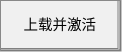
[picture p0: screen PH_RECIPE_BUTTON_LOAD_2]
VISUALIZATION PH_RECIPE_BUTTON_LOAD_2  // 122x52
VAR_IN_OUT
	RECIPE_CTRL_V2 : ST_RecipeCtrl_2;
END_VAR
    Button (0,0 120x50), "上载并激活", input disabled if: (RECIPE_CTRL_V2.sStatus.bBusy) <> 0, text list: 'TextList_Recipe', text index: 111
        p55702900: SEL(RECIPE_CTRL_V2.sCmd.bRecipeLoad, 16#000000, 16#00FF00)
        tap RECIPE_CTRL_V2.sCmd.bRecipeLoad
END_VISUALIZATION
